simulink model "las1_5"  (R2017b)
settings: Solver=ode45  StartTime=0.0  StopTime=300  MaxStep=1  RelTol=1e-3  AbsTol=1e-3
undefined symbols (not defined in the file): den, g, h0, num

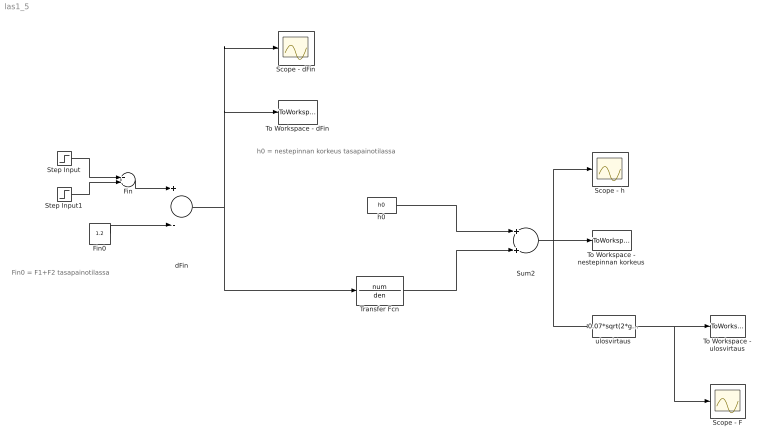
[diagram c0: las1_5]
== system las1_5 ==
  note: h0 = nestepinnan korkeus tasapainotilassa
  note: Fin0 = F1+F2 tasapainotilassa
  Fin : Sum
  Fin0 : Constant  Value=1.2
  Scope - F : Scope
  Scope - dFin : Scope
  Scope - h : Scope
  Step Input : Step  Time=10  Before=1.2  After=2.2  SampleTime=0.1
  Step Input1 : Step  Time=15  After=-1  SampleTime=0.1
  Sum2 : Sum
  To Workspace - dFin : ToWorkspace  VariableName=dFin
  To Workspace - nestepinnan korkeus : ToWorkspace  VariableName=h
  To Workspace - ulosvirtaus : ToWorkspace  VariableName=F
  Transfer Fcn : TransferFcn  Numerator=num  Denominator=den
  dFin : Sum  Inputs=+-
  h0 : Constant  Value=h0
  ulosvirtaus : Fcn  Expr=0.07*sqrt(2*g*u)
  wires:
  dFin/1 -> Transfer Fcn/1, To Workspace - dFin/1, Scope - dFin/1
  Step Input1/1 -> Fin/2
  Step Input/1 -> Fin/1
  Fin/1 -> dFin/1
  Sum2/1 -> Scope - h/1, ulosvirtaus/1, To Workspace - nestepinnan korkeus/1
  Transfer Fcn/1 -> Sum2/2
  Fin0/1 -> dFin/2
  h0/1 -> Sum2/1
  ulosvirtaus/1 -> To Workspace - ulosvirtaus/1, Scope - F/1
